| TEXAS INSTRUMENTS INCORPORATED
| Digital Light Processing Group
| IBIS Model of
| P78_1080P_HEP_S600
| This device can be powered at the following Vccs:
|  1.8 volt Vcc
| This file provides unique models under the [Model Selector] for each Vcc.
| For operation at a specific Vcc, select the appropriate model after each
| [Model Selector] keyword.
[IBIS Ver]   3.2
[Comment char]  |_char
[File Name]   dlp781ne_hep_s600.ibs
[File Rev]   1.0 | f_die
[Date]   May 24, 2022
[Source]   Data created from TI-SPICE simulations at TI-DLP.
[Notes]   The following is an IBIS list for the 0.78 4K 2xLVDS MHEP S600 DMD.
##notes##|
[Disclaimer] Property of Texas Instruments Incorporated.  Unauthorized
   reproduction and/or distribution is strictly prohibited.
   This product is protected under copyright law.
   Created  2021, (C) Copyright  2021, Texas Instruments
   Incorporated, All Rights Reserved
   UNLESS THERE IS A SIGNED, WRITTEN AGREEMENT TO THE
   CONTRARY, TEXAS INSTRUMENTS (TI) IS PROVIDING THE IBIS
   MODELS  AND WITHOUT ANY WARRANTY, EXPRESSED OR
   IMPLIED.  TI assumes no liability for:
   1) the accuracy of the IBIS models provided to your
   company;
   2) the proper functioning of these IBIS Models in your
   design or for any resulting applications; or
   3) infringement of patents, copyrights or intellectual
   property rights resulting from your use of these IBIS
   models.
   TI provides IBIS Models as a service to our customers.
   You and your company shall not distribute, sell or give
   these models to anyone else without prior written
   permission from TI.
   TI reserves the right to make changes to our products or
   to discontinue any semiconductor product or service
   without notice, and advises our customers to obtain the
   latest version of relevant information to verify, before
   placing orders, that the information being relied on is
   current.
   Please be aware that your receipt and use of the IBIS
   information provided shall serve as acceptance of these
   terms and conditions.  If you do not accept these terms,
   you should return or destroy the IBIS models and any
   other accompanying information immediately.
| Component dlp781ne_hep_s600
[Component]   dlp781ne_hep_s600
[Manufacturer]  Texas Instruments, Inc.
[Package]
|   typ   min   max
R_pkg   2.806E+00   2.110E-01   3.516E+00
L_pkg   1.157E-08   2.500E-09   1.680E-08
C_pkg   5.667E-12   3.000E-12   7.200E-12
[Pin]   signal_name   model_name   R_pin   L_pin   C_pin
P4   NO_CONNECT   NC
K4   NO_CONNECT   NC
X17   NO_CONNECT   NC
D17   NO_CONNECT   NC
E10   NO_CONNECT   NC
D6   NO_CONNECT   NC
A9   NO_CONNECT   NC
C13   NO_CONNECT   NC
B12   NO_CONNECT   NC
C17   NO_CONNECT   NC
B15   NO_CONNECT   NC
D15   NO_CONNECT   NC
E3   NO_CONNECT   NC
C7   NO_CONNECT   NC
D8   NO_CONNECT   NC
E6   NO_CONNECT   NC
C5   NO_CONNECT   NC
B8   NO_CONNECT   NC
B6   NO_CONNECT   NC
C10   NO_CONNECT   NC
E11   NO_CONNECT   NC
C6   NO_CONNECT   NC
A10   NO_CONNECT   NC
C14   NO_CONNECT   NC
B13   NO_CONNECT   NC
C16   NO_CONNECT   NC
B16   NO_CONNECT   NC
E15   NO_CONNECT   NC
D3   NO_CONNECT   NC
C8   NO_CONNECT   NC
D7   NO_CONNECT   NC
E5   NO_CONNECT   NC
C4   NO_CONNECT   NC
B9   NO_CONNECT   NC
B5   NO_CONNECT   NC
B10   NO_CONNECT   NC
W10   NO_CONNECT   NC
Z3   NO_CONNECT   NC
AA9   NO_CONNECT   NC
Y13   NO_CONNECT   NC
Z12   NO_CONNECT   NC
Y17   NO_CONNECT   NC
Z15   NO_CONNECT   NC
X15   NO_CONNECT   NC
W4   NO_CONNECT   NC
Y7   NO_CONNECT   NC
X8   NO_CONNECT   NC
Y6   NO_CONNECT   NC
X3   NO_CONNECT   NC
Z8   NO_CONNECT   NC
Z6   NO_CONNECT   NC
Z10   NO_CONNECT   NC
W11   NO_CONNECT   NC
Y3   NO_CONNECT   NC
AA10   NO_CONNECT   NC
Y14   NO_CONNECT   NC
Z13   NO_CONNECT   NC
Y16   NO_CONNECT   NC
Z16   NO_CONNECT   NC
W15   NO_CONNECT   NC
X4   NO_CONNECT   NC
Y8   NO_CONNECT   NC
X7   NO_CONNECT   NC
X6   NO_CONNECT   NC
W3   NO_CONNECT   NC
Z9   NO_CONNECT   NC
Z5   NO_CONNECT   NC
Y10   NO_CONNECT   NC
B18   D_CN<0>   INPUT_SUB_LVDS_BUF  3.515E+00  1.12E-08  6.20E-12
H24   D_CN<1>   INPUT_SUB_LVDS_BUF  3.061E+00  1.49E-08  5.70E-12
A24   D_CN<10>   INPUT_SUB_LVDS_BUF  3.053E+00  1.26E-08  5.30E-12
J26   D_CN<11>   INPUT_SUB_LVDS_BUF  3.487E+00  1.29E-08  5.60E-12
D25   D_CN<12>   INPUT_SUB_LVDS_BUF  3.060E+00  1.26E-08  5.50E-12
E23   D_CN<13>   INPUT_SUB_LVDS_BUF  3.059E+00  1.54E-08  5.90E-12
B23   D_CN<14>   INPUT_SUB_LVDS_BUF  3.059E+00  1.22E-08  5.50E-12
K24   D_CN<15>   INPUT_SUB_LVDS_BUF  3.494E+00  1.26E-08  6.30E-12
L23   D_CN<2>   INPUT_SUB_LVDS_BUF  3.059E+00  1.22E-08  6.00E-12
C18   D_CN<3>   INPUT_SUB_LVDS_BUF  3.061E+00  1.43E-08  5.90E-12
A19   D_CN<4>   INPUT_SUB_LVDS_BUF  3.513E+00  1.14E-08  5.80E-12
E24   D_CN<5>   INPUT_SUB_LVDS_BUF  3.061E+00  1.46E-08  5.70E-12
K25   D_CN<6>   INPUT_SUB_LVDS_BUF  3.060E+00  1.22E-08  5.40E-12
C26   D_CN<7>   INPUT_SUB_LVDS_BUF  3.498E+00  1.32E-08  5.60E-12
C21   D_CN<8>   INPUT_SUB_LVDS_BUF  3.059E+00  1.25E-08  5.90E-12
G25   D_CN<9>   INPUT_SUB_LVDS_BUF  3.062E+00  1.55E-08  5.30E-12
B19   D_CP<0>   INPUT_SUB_LVDS_BUF  3.513E+00  1.11E-08  6.20E-12
G24   D_CP<1>   INPUT_SUB_LVDS_BUF  3.048E+00  1.29E-08  5.80E-12
B24   D_CP<10>   INPUT_SUB_LVDS_BUF  3.053E+00  1.27E-08  5.60E-12
K26   D_CP<11>   INPUT_SUB_LVDS_BUF  3.496E+00  1.14E-08  5.70E-12
C25   D_CP<12>   INPUT_SUB_LVDS_BUF  3.060E+00  1.25E-08  5.50E-12
D23   D_CP<13>   INPUT_SUB_LVDS_BUF  3.040E+00  1.29E-08  6.00E-12
C23   D_CP<14>   INPUT_SUB_LVDS_BUF  3.058E+00  1.26E-08  5.90E-12
L24   D_CP<15>   INPUT_SUB_LVDS_BUF  3.497E+00  1.14E-08  6.40E-12
K23   D_CP<2>   INPUT_SUB_LVDS_BUF  3.058E+00  1.27E-08  6.00E-12
C19   D_CP<3>   INPUT_SUB_LVDS_BUF  3.047E+00  1.26E-08  5.90E-12
A20   D_CP<4>   INPUT_SUB_LVDS_BUF  3.512E+00  1.11E-08  5.80E-12
D24   D_CP<5>   INPUT_SUB_LVDS_BUF  3.047E+00  1.29E-08  5.90E-12
J25   D_CP<6>   INPUT_SUB_LVDS_BUF  3.059E+00  1.26E-08  5.40E-12
D26   D_CP<7>   INPUT_SUB_LVDS_BUF  3.498E+00  1.14E-08  5.70E-12
B21   D_CP<8>   INPUT_SUB_LVDS_BUF  3.048E+00  1.24E-08  5.60E-12
F25   D_CP<9>   INPUT_SUB_LVDS_BUF  3.047E+00  1.30E-08  5.40E-12
Z18   D_DN<0>   INPUT_SUB_LVDS_BUF  3.516E+00  1.13E-08  6.20E-12
T24   D_DN<1>   INPUT_SUB_LVDS_BUF  3.062E+00  1.61E-08  5.70E-12
AA24   D_DN<10>   INPUT_SUB_LVDS_BUF  3.050E+00  1.30E-08  5.20E-12
R26   D_DN<11>   INPUT_SUB_LVDS_BUF  3.497E+00  1.39E-08  5.60E-12
X25   D_DN<12>   INPUT_SUB_LVDS_BUF  3.061E+00  1.30E-08  5.50E-12
W23   D_DN<13>   INPUT_SUB_LVDS_BUF  3.062E+00  1.67E-08  5.90E-12
Z23   D_DN<14>   INPUT_SUB_LVDS_BUF  3.059E+00  1.30E-08  5.50E-12
ZP24   D_DN<15>   INPUT_SUB_LVDS_BUF  3.495E+00  1.43E-08  6.30E-12
N23   D_DN<2>   INPUT_SUB_LVDS_BUF  3.061E+00  1.28E-08  6.00E-12
Y18   D_DN<3>   INPUT_SUB_LVDS_BUF  3.053E+00  1.63E-08  5.90E-12
AA19   D_DN<4>   INPUT_SUB_LVDS_BUF  3.515E+00  1.14E-08  5.80E-12
W24   D_DN<5>   INPUT_SUB_LVDS_BUF  3.060E+00  1.60E-08  5.70E-12
P25   D_DN<6>   INPUT_SUB_LVDS_BUF  3.052E+00  1.30E-08  5.40E-12
Y26   D_DN<7>   INPUT_SUB_LVDS_BUF  3.487E+00  1.46E-08  5.60E-12
Y21   D_DN<8>   INPUT_SUB_LVDS_BUF  3.061E+00  1.30E-08  5.90E-12
U25   D_DN<9>   INPUT_SUB_LVDS_BUF  3.061E+00  1.68E-08  5.30E-12
Z19   D_DP<0>   INPUT_SUB_LVDS_BUF  3.514E+00  1.08E-08  6.20E-12
U24   D_DP<1>   INPUT_SUB_LVDS_BUF  3.051E+00  1.21E-08  5.80E-12
Z24   D_DP<10>   INPUT_SUB_LVDS_BUF  3.050E+00  1.20E-08  5.60E-12
P26   D_DP<11>   INPUT_SUB_LVDS_BUF  3.499E+00  1.11E-08  5.80E-12
Y25   D_DP<12>   INPUT_SUB_LVDS_BUF  3.051E+00  1.21E-08  5.50E-12
X23   D_DP<13>   INPUT_SUB_LVDS_BUF  3.048E+00  1.21E-08  5.90E-12
Y23   D_DP<14>   INPUT_SUB_LVDS_BUF  3.057E+00  1.19E-08  5.90E-12
N24   D_DP<15>   INPUT_SUB_LVDS_BUF  3.497E+00  1.11E-08  6.40E-12
P23   D_DP<2>   INPUT_SUB_LVDS_BUF  3.050E+00  1.19E-08  5.90E-12
Y19   D_DP<3>   INPUT_SUB_LVDS_BUF  3.048E+00  1.19E-08  5.90E-12
AA20   D_DP<4>   INPUT_SUB_LVDS_BUF  3.514E+00  1.09E-08  5.80E-12
X24   D_DP<5>   INPUT_SUB_LVDS_BUF  3.039E+00  1.21E-08  5.80E-12
R25   D_DP<6>   INPUT_SUB_LVDS_BUF  3.051E+00  1.20E-08  5.40E-12
X26   D_DP<7>   INPUT_SUB_LVDS_BUF  3.488E+00  1.10E-08  5.70E-12
Z21   D_DP<8>   INPUT_SUB_LVDS_BUF  3.051E+00  1.21E-08  5.60E-12
V25   D_DP<9>   INPUT_SUB_LVDS_BUF  3.046E+00  1.20E-08  5.30E-12
B3   NO_CONNECT   NC
C3   NO_CONNECT   NC
Y4   NO_CONNECT   NC
Y5   NO_CONNECT   NC
H23   DCLK_CN   INPUT_SUB_LVDS_BUF  3.060E+00  1.19E-08  6.00E-12
G23   DCLK_CP   INPUT_SUB_LVDS_BUF  3.059E+00  1.22E-08  6.00E-12
T23   DCLK_DN   INPUT_SUB_LVDS_BUF  3.051E+00  1.24E-08  6.00E-12
U23   DCLK_DP   INPUT_SUB_LVDS_BUF  3.049E+00  1.19E-08  6.00E-12
E14   NO_CONNECT   NC   2.110E-01  3.20E-09  3.60E-12
D13   NO_CONNECT   NC   3.960E-01  3.80E-09  3.40E-12
W13   NO_CONNECT   NC   5.440E-01  4.60E-09  4.10E-12
Y12   NO_CONNECT   NC   7.350E-01  9.20E-09  3.70E-12
W12   NO_CONNECT   NC   6.250E-01  4.50E-09  4.30E-12
Y11   NO_CONNECT   NC   8.190E-01  6.80E-09  4.00E-12
Y15   NO_CONNECT   NC   4.990E-01  4.30E-09  3.40E-12
E13   NO_CONNECT   NC   5.350E-01  5.50E-09  4.00E-12
C12   NO_CONNECT   NC   7.300E-01  7.70E-09  3.70E-12
E12   NO_CONNECT   NC   6.810E-01  5.80E-09  4.30E-12
C11   NO_CONNECT   NC   8.140E-01  6.00E-09  4.00E-12
D16   NO_CONNECT   NC   2.870E-01  4.10E-09  3.20E-12
C15   NO_CONNECT   NC   3.850E-01  4.70E-09  3.00E-12
W14   NO_CONNECT   NC   2.110E-01  2.50E-09  3.60E-12
X13   NO_CONNECT   NC   4.010E-01  4.50E-09  3.40E-12
W18   NO_CONNECT   NC
G4   PWRDNZ   INPUT_BUF   1.639E+00  6.30E-09  4.60E-12
G3   NO_CONNECT   NC
U2   SCPCLK   INPUT_BUF   1.180E+00  7.60E-09  4.30E-12
T3   SCPDI   INPUT_BUF   2.406E+00  1.04E-08  5.10E-12
U3   SCPDO   INPUT_BUF   1.053E+00  6.70E-09  4.40E-12
U4   SCPENZ   INPUT_BUF   1.803E+00  7.60E-09  4.80E-12
E4   NO_CONNECT   NC
D4   NO_CONNECT   NC
W5   NO_CONNECT   NC
W6   NO_CONNECT   NC
F26   SCTRL_CN   INPUT_SUB_LVDS_BUF  3.496E+00  1.26E-08  5.60E-12
G26   SCTRL_CP   INPUT_SUB_LVDS_BUF  3.499E+00  1.12E-08  5.70E-12
V26   SCTRL_DN   INPUT_SUB_LVDS_BUF  3.486E+00  1.36E-08  5.60E-12
U26   SCTRL_DP   INPUT_SUB_LVDS_BUF  3.499E+00  1.09E-08  5.70E-12
W16   NO_CONNECT   NC   1.162E+00  8.10E-09  5.40E-12
W17   NO_CONNECT   NC   1.029E+00  6.80E-09  5.90E-12
H3   NO_CONNECT   NC   1.152E+00  8.80E-09  4.60E-12
G2   NO_CONNECT   NC   2.499E+00  9.70E-09  4.90E-12
F3   NO_CONNECT   NC   1.111E+00  8.50E-09  4.50E-12
A5   VCC   POWER
A6   VCC   POWER
B2   VCC   POWER
C1   VCC   POWER
D10   VCC   POWER
D12   VCC   POWER
D19   VCC   POWER
D22   VCC   POWER
E8   VCC   POWER
E19   VCC   POWER
E20   VCC   POWER
E21   VCC   POWER
E22   VCC   POWER
F1   VCC   POWER
F2   VCC   POWER
J2   VCC   POWER
K1   VCC   POWER
L1   VCC   POWER
L25   VCC   POWER
M3   VCC   POWER
M4   VCC   POWER
M25   VCC   POWER
N1   VCC   POWER
N25   VCC   POWER
P1   VCC   POWER
R2   VCC   POWER
V1   VCC   POWER
V2   VCC   POWER
W8   VCC   POWER
W19   VCC   POWER
W20   VCC   POWER
W21   VCC   POWER
W22   VCC   POWER
X10   VCC   POWER
X12   VCC   POWER
X19   VCC   POWER
X22   VCC   POWER
Y1   VCC   POWER
Z1   VCC   POWER
Z2   VCC   POWER
AA2   VCC   POWER
AA5   VCC   POWER
AA6   VCC   POWER
A3   VCC2   POWER
A4   VCC2   POWER
A25   VCC2   POWER
B26   VCC2   POWER
L26   VCC2   POWER
M26   VCC2   POWER
N26   VCC2   POWER
Z26   VCC2   POWER
AA3   VCC2   POWER
AA4   VCC2   POWER
AA25   VCC2   POWER
A7   VCCI   POWER
A8   VCCI   POWER
A11   VCCI   POWER
A16   VCCI   POWER
A17   VCCI   POWER
A18   VCCI   POWER
A21   VCCI   POWER
A22   VCCI   POWER
A23   VCCI   POWER
AA7   VCCI   POWER
AA8   VCCI   POWER
AA11   VCCI   POWER
AA16   VCCI   POWER
AA17   VCCI   POWER
AA18   VCCI   POWER
AA21   VCCI   POWER
AA22   VCCI   POWER
AA23   VCCI   POWER
B4   VSS   GND
B7   VSS   GND
B11   VSS   GND
B14   VSS   GND
B17   VSS   GND
B20   VSS   GND
B22   VSS   GND
B25   VSS   GND
C2   VSS   GND
C9   VSS   GND
C20   VSS   GND
C22   VSS   GND
C24   VSS   GND
D1   VSS   GND
D2   VSS   GND
D5   VSS   GND
D9   VSS   GND
D11   VSS   GND
D14   VSS   GND
D18   VSS   GND
D20   VSS   GND
D21   VSS   GND
E1   VSS   GND
E2   VSS   GND
E7   VSS   GND
E9   VSS   GND
E16   VSS   GND
E17   VSS   GND
E18   VSS   GND
E25   VSS   GND
E26   VSS   GND
F4   VSS   GND
F23   VSS   GND
F24   VSS   GND
H2   VSS   GND
H4   VSS   GND
H25   VSS   GND
H26   VSS   GND
J23   VSS   GND
J24   VSS   GND
K2   VSS   GND
L2   VSS   GND
L3   VSS   GND
L4   VSS   GND
M1   VSS   GND
M2   VSS   GND
M23   VSS   GND
M24   VSS   GND
N2   VSS   GND
N3   VSS   GND
N4   VSS   GND
P2   VSS   GND
R23   VSS   GND
R24   VSS   GND
T2   VSS   GND
T4   VSS   GND
T25   VSS   GND
T26   VSS   GND
V4   VSS   GND
V23   VSS   GND
V24   VSS   GND
W1   VSS   GND
W2   VSS   GND
W7   VSS   GND
W9   VSS   GND
W25   VSS   GND
W26   VSS   GND
X1   VSS   GND
X2   VSS   GND
X5   VSS   GND
X9   VSS   GND
X11   VSS   GND
X14   VSS   GND
X18   VSS   GND
X20   VSS   GND
X21   VSS   GND
Y2   VSS   GND
Y9   VSS   GND
Y20   VSS   GND
Y22   VSS   GND
Y24   VSS   GND
Z4   VSS   GND
Z7   VSS   GND
Z11   VSS   GND
Z14   VSS   GND
Z17   VSS   GND
Z20   VSS   GND
Z22   VSS   GND
Z25   VSS   GND
G1   N/C   NC
H1   N/C   NC
J1   N/C   NC
J3   N/C   NC
J4   N/C   NC
K3   N/C   NC
P3   N/C   NC
R1   N/C   NC
R3   N/C   NC
R4   N/C   NC
T1   N/C   NC
U1   N/C   NC
V3   N/C   NC
X16   N/C   NC
| NOTE:  The [Diff Pin] section may get flagged by early versions of the
|   ibischk program
[Diff Pin]  inv_pin   vdiff   tdelay_typ
B19   B18   200mv   NA
G24   H24   200mv   NA
B24   A24   200mv   NA
K26   J26   200mv   NA
C25   D25   200mv   NA
D23   E23   200mv   NA
C23   B23   200mv   NA
L24   K24   200mv   NA
K23   L23   200mv   NA
C19   C18   200mv   NA
A20   A19   200mv   NA
D24   E24   200mv   NA
J25   K25   200mv   NA
D26   C26   200mv   NA
B21   C21   200mv   NA
F25   G25   200mv   NA
Z19   Z18   200mv   NA
U24   T24   200mv   NA
Z24   AA24   200mv   NA
P26   R26   200mv   NA
Y25   X25   200mv   NA
X23   W23   200mv   NA
Y23   Z23   200mv   NA
N24   ZP24   200mv   NA
P23   N23   200mv   NA
Y19   Y18   200mv   NA
AA20   AA19   200mv   NA
X24   W24   200mv   NA
R25   P25   200mv   NA
X26   Y26   200mv   NA
Z21   Y21   200mv   NA
V25   U25   200mv   NA
G23   H23   200mv   NA
U23   T23   200mv   NA
G26   F26   200mv   NA
U26   V26   200mv   NA
| Model INPUT_SUB_LVDS_BUF
[Model Selector]   INPUT_SUB_LVDS_BUF
INPUT_SUBLVDS_BUF_18   1.8 volt Vcc
| Model INPUT_BUF
[Model Selector]   INPUT_BUF
INPUT_BUF_18   1.8 volt Vcc
| Model OUTPUT_BUF
[Model Selector]   OUTPUT_BUF
OUTPUT_BUF_18   1.8 volt Vcc
| Models and submodels in the file (3): INPUT_SUBLVDS_BUF_18 (Input), INPUT_BUF_18 (Input), OUTPUT_BUF_18 (Output)
